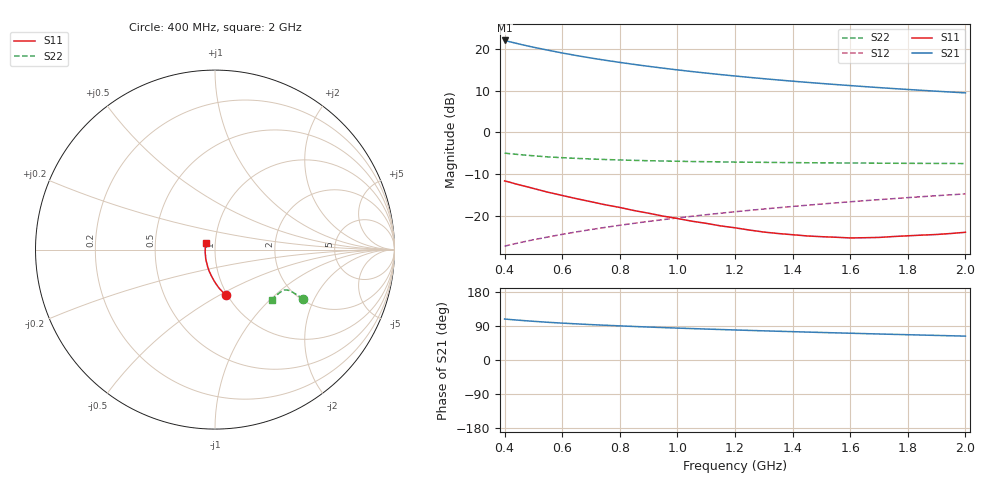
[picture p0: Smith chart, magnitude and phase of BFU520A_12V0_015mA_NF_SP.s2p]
! Filename:  P:\Prog\Test\Noise\ATS_data\Testdata_Net\06 Compressed Noise after Statistics\BFU520A_APG2013_30_A05_12p0V_015mA_NF_CM01_D.sf
! Date/Time: Wed 24/Apr/2013 20:06:22
! BFU520A_APG2013_30_A05_12p0V_1to20mA_NF_CM01_Bias7_R.sf
! Noise Parameter Data File
! BFU520A_APG2013_30_A05_12p0V_1to20mA_NF_CM01
! Date/time: Thu Apr 11 10:46:45 2013
! VAR V_out= 12.001000
! VAR I_out= 14.995000
! VAR V_in= 0.805700
! VAR I_in= 0.151200
! Device data file deembeded for feedlines and parallel
! Original file: \06 Compressed Noise after Statistics\BFU520A_APG2013_30_A05_12p0V_015mA_NF_CM01_R.sf
! Feed-files: PR017V01_150413_Feed1.s2p, PR017V01_150413_Feed2.s2p
! Parallel-file: PR017V01_150413_Par.s2p
# MHz S MA R 50
!  Freq-MHz  S11-mag  S11-arg  S21-mag  S21-arg  S12-mag  S12-arg  S22-mag  S22-arg
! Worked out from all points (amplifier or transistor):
!   37 points, 400 MHz to 2 GHz, reference 50 ohm
!   highest |S21| = 22.0 dB at 400 MHz (marker M1)
!   |S21| within 3 dB of that: start of sweep to 599.7 MHz
!   unconditionally stable (mu >= 1): 1.193 GHz to end of sweep
!   at 500 MHz: K = 0.88, MSG = 23.1 dB, |S12| = -25.8 dB
!   at 1.1 GHz: K = 1.00, MSG = 17.0 dB, |S12| = -19.8 dB
!   at 2 GHz: K = 1.00, MAG = 11.8 dB, |S12| = -14.8 dB
!   lowest NFmin = 1.03 dB at 460 MHz
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400  0.2615 -76.4  12.64 108.2  0.04308 71.6  0.5633 -29.0
420  0.2508 -78.2  12.15 106.8  0.04476 71.7  0.5536 -29.0
440  0.2397 -79.9  11.69 105.5  0.04643 71.8  0.5452 -29.0
460  0.2301 -81.3  11.26 104.4  0.04807 72.0  0.5373 -29.0
480  0.2213 -83.0  10.86 103.2  0.04974 72.1  0.5295 -29.0
500  0.2122 -84.6  10.49 102.1  0.0514 72.2  0.5231 -29.0
550  0.1914 -88.2  9.673 99.5  0.05547 72.5  0.5073 -28.8
600  0.1749 -91.5  8.945 97.3  0.05973 72.8  0.4963 -28.8
650  0.1599 -94.7  8.329 95.3  0.06391 73.0  0.4866 -28.8
700  0.147 -98.1  7.789 93.4  0.06817 73.2  0.4787 -28.8
750  0.1351 -101.3  7.312 91.7  0.07244 73.3  0.4718 -28.9
800  0.1255 -104.8  6.896 90.0  0.07673 73.4  0.466 -29.1
850  0.1152 -108.2  6.521 88.5  0.08101 73.4  0.4607 -29.2
950  0.09883 -115.3  5.882 85.6  0.08962 73.4  0.4527 -29.8
1050  0.08589 -122.8  5.359 82.9  0.0983 73.3  0.4465 -30.4
1150  0.07545 -132.1  4.926 80.5  0.1071 73.1  0.4415 -31.1
1200  0.07155 -136.2  4.735 79.3  0.1115 73.0  0.4394 -31.6
1350  0.06107 -151.2  4.245 75.8  0.1246 72.5  0.4347 -33.0
1500  0.05598 -168.6  3.854 72.7  0.1379 71.8  0.4301 -34.6
1650  0.0544 175.6  3.534 69.6  0.1513 71.1  0.4277 -36.5
1750  0.05622 165.2  3.348 67.7  0.1601 70.6  0.4251 -37.8
2000  0.06324 145.0  2.972 63.0  0.1825 69.1  0.4221 -41.3
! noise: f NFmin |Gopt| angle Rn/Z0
400  1.076  0.07613  -158.7  0.1171
460  1.034  0.08662  -159  0.1147
600  1.17  0.05703  -133.6  0.1371
800  1.123  0.1257  -153.6  0.104
1000  1.126  0.1265  -149  0.107
1200  1.145  0.139  -141.1  0.1163
1400  1.193  0.1674  -134.5  0.1101
1600  1.177  0.1651  -134.2  0.1139
1800  1.172  0.2151  -133.1  0.104
2000  1.192  0.2117  -126.7  0.1167
